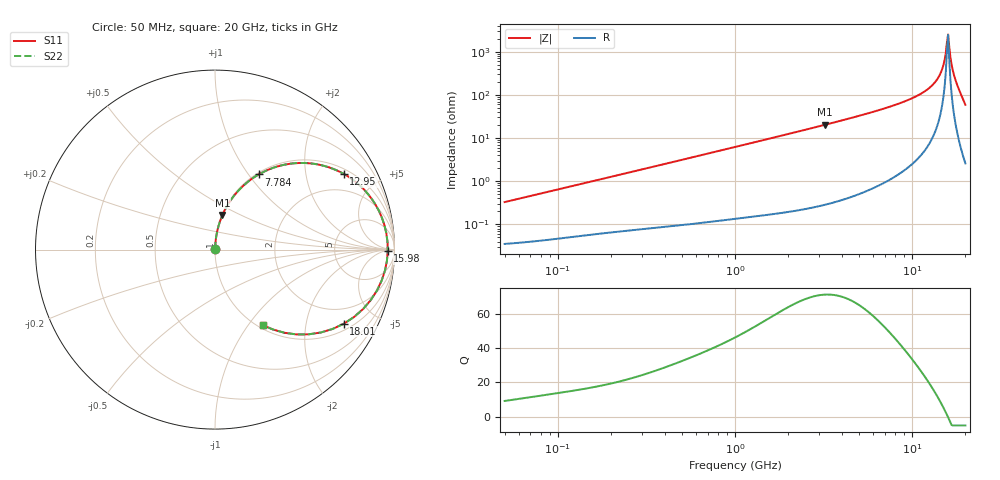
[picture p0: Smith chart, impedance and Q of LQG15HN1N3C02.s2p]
!Murata Part Number: LQG15HN1N3C02
!These Parameters are Measured in Series Mode Connection
!  o--[Z]--o
!Port1  Port2
!  o-------o
!Freq. Start=50[MHz] Stop=20[GHz], 401[Steps]
# Hz S RI R 50
!Freq.(Hz) S11(Real) S11(Imag) S21(Real) S21(Imag) S12(Real) S12(Imag) S22(Real) S22(Imag)
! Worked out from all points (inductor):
!   401 points, 50 MHz to 20 GHz, reference 50 ohm
!   read as one part in series: L = 1.03 nH near 51.52 MHz
!   highest Q = 71.1 at 3.217 GHz (marker M1), where L = 998 pH
!   self-resonance near 15.74 GHz
!   S11 on the Smith chart (normalised r, x): 50 MHz: 1.00, +0.01; 7.784 GHz: 1.02, +1.12; 12.95 GHz: 1.19, +3.27; 15.98 GHz: 50, -11; 18.01 GHz: 1.26, -3.30; 20 GHz: 1.05, -1.17
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5e7  0.000363 0.00326  0.9996 -0.00326  0.9996 -0.00326  0.000363 0.00326
1.364002e8  0.000618 0.0087  0.9994 -0.0087  0.9994 -0.0087  0.000618 0.0087
3.721004e8  0.00138 0.0232  0.9986 -0.0232  0.9986 -0.0232  0.00138 0.0232
1e9  0.00513 0.0614  0.9949 -0.0614  0.9949 -0.0614  0.00513 0.0614
2.728004e9  0.0303 0.1645  0.9697 -0.1645  0.9697 -0.1645  0.0303 0.1645
3.216634e9  0.0416 0.1929  0.9584 -0.1929  0.9584 -0.1929  0.0416 0.1929
5.194772e9  0.1069 0.3013  0.8931 -0.3013  0.8931 -0.3013  0.1069 0.3013
7.442007e9  0.2215 0.4052  0.7785 -0.4052  0.7785 -0.4052  0.2215 0.4052
7.784049e9  0.243 0.4184  0.757 -0.4184  0.757 -0.4184  0.243 0.4184
1.019291e10  0.4289 0.4797  0.5711 -0.4797  0.5711 -0.4797  0.4289 0.4797
1.295331e10  0.7176 0.4218  0.2824 -0.4218  0.2824 -0.4218  0.7176 0.4218
1.396067e10  0.831 0.3337  0.169 -0.3337  0.169 -0.3337  0.831 0.3337
1.460232e10  0.8949 0.2495  0.1051 -0.2495  0.1051 -0.2495  0.8949 0.2495
1.504638e10  0.9302 0.1772  0.0698 -0.1772  0.0698 -0.1772  0.9302 0.1772
1.550395e10  0.9546 0.0909  0.0454 -0.0909  0.0454 -0.0909  0.9546 0.0909
1.573793e10  0.961 0.0428  0.039 -0.0428  0.039 -0.0428  0.961 0.0428
1.597544e10  0.9624 -0.00831  0.0376 0.00831  0.0376 0.00831  0.9624 -0.00831
1.621653e10  0.958 -0.0618  0.042 0.0618  0.042 0.0618  0.958 -0.0618
1.721783e10  0.8677 -0.2814  0.1323 0.2814  0.1323 0.2814  0.8677 -0.2814
1.800918e10  0.7179 -0.4127  0.2821 0.4127  0.2821 0.4127  0.7179 -0.4127
1.88369e10  0.5212 -0.4721  0.4788 0.4721  0.4788 0.4721  0.5212 -0.4721
2e10  0.2655 -0.4202  0.7345 0.4202  0.7345 0.4202  0.2655 -0.4202
